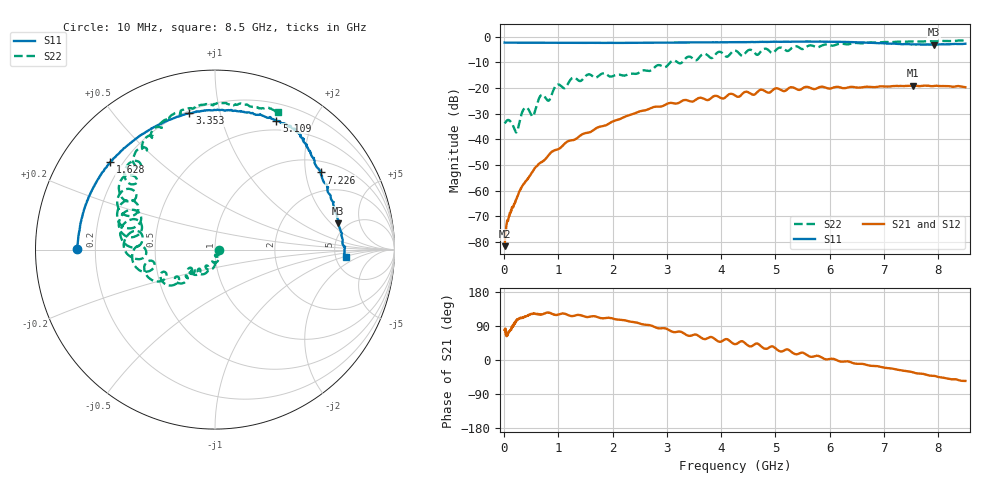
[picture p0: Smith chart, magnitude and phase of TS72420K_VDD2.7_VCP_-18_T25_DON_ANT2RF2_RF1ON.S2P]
!Agilent Technologies,E5071C,MY46417908,A.11.23
!Date: Thu Oct 03 16:40:38 2019
!Data & Calibration Information:
!Freq	S11:SOLT2(ON)	S21:SOLT2(ON)	S12:SOLT2(ON)	S22:SOLT2(ON)
!PortZ  Port1:50+j0  Port2:50+j0
!Above PortZ is port z conversion or system Z0 setting when saving the data.
!When reading, reference impedance value at option line is always used.
# Hz S dB R 50
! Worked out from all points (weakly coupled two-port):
!   1601 points, 10 MHz to 8.5 GHz, reference 50 ohm
!   highest |S21| = -19.02 dB at 7.54 GHz (marker M1); lowest = -81.6 dB at 10 MHz (marker M2)
!   lowest |S11| = -3.1 dB at 7.922 GHz (marker M3), VSWR 5.71, Z = 213 + j122 ohm
!   |S11| at or under -10 dB: nowhere
!   |S22| runs from -37.3 to -1.5 dB; largest |S21 - S12| = 0.0014
!   S11 on the Smith chart (normalised r, x): 10 MHz: 0.13, +0.00; 1.628 GHz: 0.15, +0.36; 3.353 GHz: 0.21, +0.81; 5.109 GHz: 0.39, +1.51; 7.226 GHz: 1.33, +2.43; 8.5 GHz: 6.22, -1.14
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1e7  -2.29 179.8  -81.63 79.5  -85.12 56.1  -33.76 0.0
8.42875e7  -2.32 177.7  -70.47 75.7  -70.11 73.9  -32.50 -25.4
2.2225e8  -2.34 174.1  -63.45 102.6  -63.57 102.3  -37.29 -47.9
3.761312e8  -2.35 170.1  -56.95 114.6  -57.01 115.2  -27.84 -59.8
5.512375e8  -2.35 165.7  -51.75 122.9  -51.74 122.9  -30.39 -66.9
6.838938e8  -2.36 162.4  -48.97 120.2  -48.97 119.3  -22.73 -86.4
8.1655e8  -2.35 159.1  -46.27 124.7  -46.32 124.9  -24.93 -100.2
9.757375e8  -2.37 155.2  -43.99 118.8  -44.04 118.6  -18.69 -105.1
1.426769e9  -2.39 144.8  -38.20 117.5  -38.20 117.2  -17.05 -125.4
1.628406e9  -2.38 140.1  -36.69 115.4  -36.66 115.4  -15.36 -138.8
2.434956e9  -2.39 121.0  -29.63 99.0  -29.57 98.9  -14.47 -136.2
2.843538e9  -2.33 111.5  -27.26 83.7  -27.21 83.7  -11.04 -140.2
3.352938e9  -2.24 100.6  -24.67 66.7  -24.64 66.9  -8.26 -153.5
4.255e9  -2.13 81.4  -22.89 41.8  -22.88 42.0  -5.41 168.1
4.377044e9  -2.12 78.8  -22.56 49.7  -22.59 50.0  -7.41 162.6
5.109306e9  -1.98 64.6  -20.83 22.5  -20.81 22.5  -4.26 148.3
5.671769e9  -1.93 57.5  -20.19 8.3  -20.17 8.5  -3.43 133.2
7.088538e9  -2.73 39.3  -19.42 -21.8  -19.47 -21.7  -2.10 105.0
7.2265e9  -2.75 36.1  -19.19 -24.9  -19.24 -25.1  -1.95 103.5
7.539569e9  -2.97 25.2  -19.02 -32.8  -19.02 -33.3  -1.84 95.7
7.921619e9  -3.07 12.0  -19.22 -41.9  -19.12 -42.0  -1.82 83.5
8.5e9  -2.72 -3.3  -19.67 -55.3  -19.75 -55.3  -1.48 65.4
